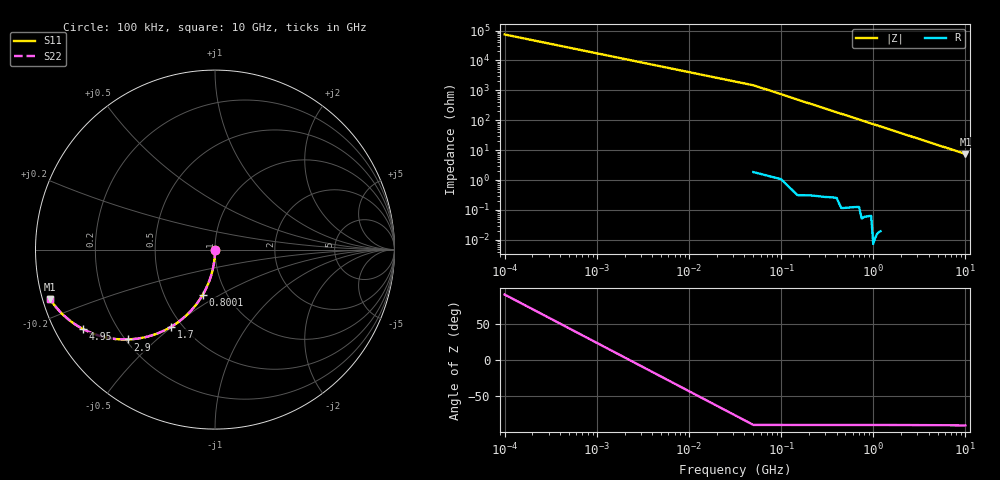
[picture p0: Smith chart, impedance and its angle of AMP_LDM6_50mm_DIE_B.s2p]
! Created Tue Aug  7 13:44:51 2007
# hz S ri R 50
! 2 Port Network Data from SP1.SP block
! freq  reS11  imS11  reS21  imS21  reS12  imS12  reS22  imS22
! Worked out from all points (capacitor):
!   201 points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, 100 kHz to 10 GHz, reference 50 ohm
!   read as one part in shunt: C = 2.15 pF near 50.1 MHz
!   lowest |Z| = 7.49 ohm at 10 GHz (marker M1)
!   S11 on the Smith chart (normalised r, x): 100 kHz: 1.00, +0.00; 800.1 MHz: 0.78, -0.42; 1.7 GHz: 0.43, -0.50; 2.9 GHz: 0.21, -0.41; 4.95 GHz: 0.08, -0.28; 10 GHz: 0.02, -0.15
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100000  6.3e-06 0.000291  1 0.000337  1 0.000337  4.46e-06 0.00039
5.01e7  -0.00029 -0.0167  0.9997 -0.017  0.9997 -0.017  -0.00029 -0.017
1.001e8  -0.00115 -0.0331  0.9988 -0.0336  0.9988 -0.0336  -0.00115 -0.0336
1.501e8  -0.00258 -0.0511  0.9974 -0.0505  0.9974 -0.0505  -0.00258 -0.0504
2.001e8  -0.00456 -0.0674  0.9954 -0.0671  0.9954 -0.0671  -0.00457 -0.067
2.501e8  -0.00709 -0.0837  0.9929 -0.0836  0.9929 -0.0836  -0.0071 -0.0835
3.001e8  -0.0102 -0.0999  0.9898 -0.1001  0.9898 -0.1001  -0.0102 -0.0999
4.001e8  -0.0179 -0.1315  0.982 -0.1323  0.982 -0.1323  -0.0179 -0.1321
5.501e8  -0.0332 -0.1788  0.9667 -0.179  0.9667 -0.179  -0.0332 -0.1787
8.001e8  -0.0676 -0.2509  0.9322 -0.251  0.9322 -0.251  -0.0676 -0.2506
1.0001e9  -0.1016 -0.3025  0.8981 -0.3024  0.8981 -0.3024  -0.1017 -0.3019
1.2501e9  -0.15 -0.3576  0.8497 -0.3575  0.8497 -0.3575  -0.15 -0.3569
1.7001e9  -0.2459 -0.4303  0.7538 -0.4313  0.7538 -0.4313  -0.2458 -0.4306
2.3001e9  -0.3737 -0.4848  0.6259 -0.4849  0.6259 -0.4849  -0.3736 -0.4841
2.9001e9  -0.487 -0.5007  0.5126 -0.5014  0.5126 -0.5014  -0.4867 -0.5006
3.3501e9  -0.5591 -0.498  0.4406 -0.4984  0.4406 -0.4984  -0.5586 -0.4975
4.1001e9  -0.6554 -0.4773  0.3442 -0.4776  0.3442 -0.4776  -0.6549 -0.4766
4.9501e9  -0.7352 -0.4435  0.2644 -0.4439  0.2644 -0.4439  -0.7347 -0.4428
5.0001e9  -0.7391 -0.4411  0.2605 -0.4419  0.2605 -0.4419  -0.7385 -0.4408
6.7001e9  -0.8362 -0.3718  0.1632 -0.3737  0.1632 -0.3737  -0.8357 -0.3725
8.3501e9  -0.8886 -0.3174  0.1108 -0.3193  0.1108 -0.3193  -0.888 -0.3179
1.00001e10  -0.9201 -0.2745  0.0792 -0.2766  0.0792 -0.2766  -0.9195 -0.275
